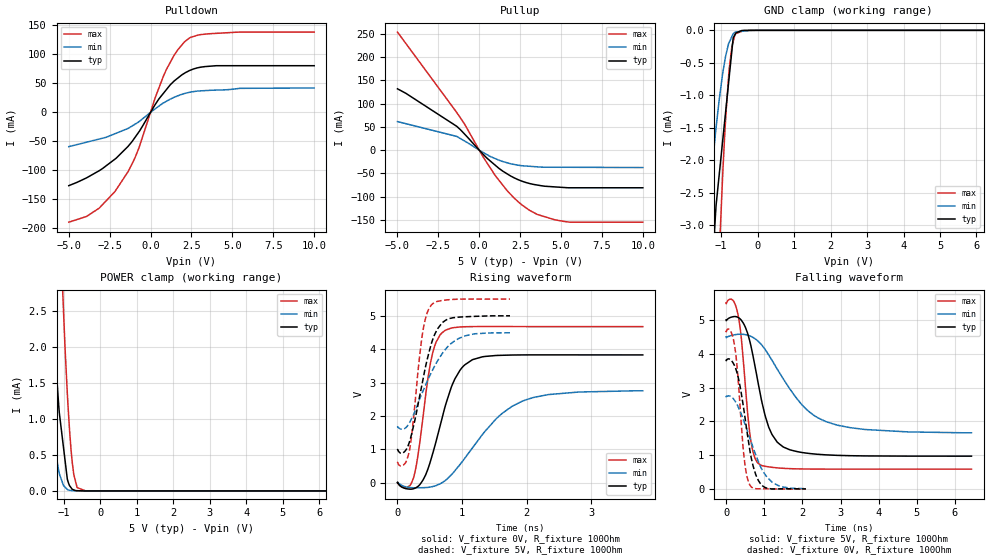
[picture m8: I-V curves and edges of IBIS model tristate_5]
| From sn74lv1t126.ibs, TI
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|   tristate_5 Model
[Model]   tristate_5
Model_type   3-state
Polarity   Non-Inverting
Vmeas = 2.5
Vref = 0
Cref = 30pF
Rref = 100
|   typ   min   max
|   (nom PVT)   (fast PVT)   (slow PVT)
C_comp   2.245e-12   2.225e-12   2.269e-12
| Where nom  PVT is Nominal Process, 5V, 40C
|   Fast PVT is Strong Process,  5.5V, -40C
|   Slow PVT is Weak Process,   4.5V, 140C
[Voltage Range]   5   4.5   5.5
|Junction Temperature
[Temperature Range]   40   140   -40
[Pullup Reference]   5   4.5   5.5
[Pulldown Reference]   0   0   0
[Power Clamp Reference]   5   4.5   5.5
[GND Clamp Reference]   0   0   0
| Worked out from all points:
|   slope of the pulldown table from 0 to 0.75 V, typ, clamps not added: 23.8 ohm
|   slope of the pullup table from 0 to 0.75 V, typ, clamps not added: 29.4 ohm
|   GND clamp passes 1 mA (typ) near -0.83 V on its own axis
|   POWER clamp passes 1 mA (typ) near -1.10 V on its own axis
|   falling waveform, V_fixture 5V, R_fixture 100Ohm: 20-80 % time 480ps typ, 1.11ns min, 237ps max; typ from 5 V to 0.975 V
|   rising waveform, V_fixture 0V, R_fixture 100Ohm: 20-80 % time 348ps typ, 740ps min, 202ps max; typ from 0 V to 3.83 V
|   rising waveform, V_fixture 5V, R_fixture 100Ohm: 20-80 % time 270ps typ, 425ps min, 163ps max; typ from 0.975 V to 5 V
|   falling waveform, V_fixture 0V, R_fixture 100Ohm: 20-80 % time 328ps typ, 548ps min, 195ps max; typ from 3.83 V to 0.009 V
[Pulldown]
|   Voltage   I(typ)   I(min)   I(max)
-5V       -126.6mA   -59.23mA   -189.6mA
-3.905V   -113mA     -51.53mA   -179.6mA
-3.14V    -100.8mA   -46.15mA   -165.3mA
-2.189V   -81.04mA   -37.15mA   -137mA
-1.375V   -58.76mA   -27.86mA   -102.5mA
-709.5mV  -33.68mA   -16.18mA   -61.28mA
302.5mV   14.21mA    6.321mA    26.75mA
803mV     33.33mA    16.31mA    63.51mA
1.419V    53.33mA    25.57mA    97.38mA
2.145V    68.57mA    32.8mA     123.1mA
3.547V    79.25mA    37.69mA    135.4mA
10V       80.29mA    41.89mA    138.3mA
[GND Clamp]
|   Voltage   I(typ)   I(min)   I(max)
-5V       -79.76mA   -44.68mA   -116.9mA
-1.375V   -5.076mA   -2.914mA   -8.957mA
-1.255V   -3.79mA    -2.182mA   -6.711mA
-1.157V   -2.846mA   -1.586mA   -5.027mA
-1.05V    -2.206mA   -1.056mA   -3.423mA
-963mV    -1.726mA   -683.2uA   -2.291mA
-877.5mV  -1.256mA   -396.8uA   -1.369mA
-786.5mV  -756.1uA   -193.2uA   -640.4uA
-704mV    -303uA     -93.82uA   -242.6uA
-670mV    -116.2uA   -53.23uA   -171.9uA
-616.5mV  -62.01uA   -27.22uA   -60.64uA
10V       0A         0A         0A
[Pullup]
|   Voltage   I(typ)   I(min)   I(max)
-5V       132mA      61.56mA    253.9mA
-4.5V     122.6mA    57.15mA    230.1mA
-1.375V   51.32mA    29.6mA     81.04mA
-858mV    33.19mA    18.98mA    53.77mA
265mV     -9.864mA   -5.349mA   -15.98mA
968mV     -32.02mA   -17.94mA   -53.99mA
1.788V    -52.63mA   -27.86mA   -90.19mA
2.635V    -66.91mA   -33.47mA   -118.3mA
3.547V    -74.93mA   -35.76mA   -138.1mA
4.631V    -78.93mA   -36.67mA   -149.7mA
5.192V    -80.23mA   -36.69mA   -153.2mA
10V       -80.78mA   -37.35mA   -154.8mA
[POWER Clamp]
|   Voltage   I(typ)   I(min)   I(max)
-5V       81.69mA    45.06mA    132.8mA
-1.735V   7.225mA    3.528mA    16.16mA
-1.373V   3.058mA    1.094mA    8.26mA
-1.27V    2.158mA    682.3uA    6.386mA
-1.125V   1.09mA     243.3uA    4.061mA
-1.067V   846.4uA    157.9uA    3.223mA
-1.008V   598.9uA    73.93uA    2.494mA
-850.5mV  81.54uA    9.359uA    905.1uA
-726mV    14.49uA    3.161uA    225.7uA
-632.5mV  3.405uA    656.9nA    46.34uA
-401.5mV  48.63nA    305.4nA    305.7nA
10V       0A         0A         0A
[Ramp]
R_load = 100
|   typ   min   max
dV/dt_r   2.29631/3.48301e-10   1.65453/7.38171e-10   2.80548/2.01165e-10
dV/dt_f   2.41476/4.76742e-10   1.70472/1.10947e-09   2.94472/2.36728e-10
[Falling Waveform]
V_fixture = 5V
V_fixture_min = 4.5V
V_fixture_max = 5.5V
R_fixture = 100Ohm
|   Time   V(typ)   V(min)   V(max)
0s        5V         4.5V       5.5V
172ps     5.09V      4.549V     5.585V
314ps     5.074V     4.574V     5.147V
640ps     4.282V     4.517V     1.49V
902ps     2.774V     4.299V     717.3mV
1.114ns   1.84V      3.967V     659.6mV
1.338ns   1.392V     3.55V      630.3mV
2.018ns   1.079V     2.457V     597.1mV
2.604ns   1.015V     2.001V     592.9mV
6.434ns   975.5mV    1.665V     592.1mV
[Rising Waveform]
V_fixture = 0V
V_fixture_min = 0V
V_fixture_max = 0V
R_fixture = 100Ohm
|   Time   V(typ)   V(min)   V(max)
0s        997pV      9.968nV    1.769nV
146ps     -188mV     -136.3mV   -148.9mV
250ps     -184.7mV   -156.4mV   148.6mV
518ps     687.7mV    -130.8mV   3.652V
598ps     1.236V     -90.43mV   4.212V
736ps     2.268V     54.71mV    4.559V
1.044ns   3.532V     733.4mV    4.672V
1.538ns   3.811V     1.93V      4.678V
1.92ns    3.827V     2.43V      4.677V
3.798ns   3.827V     2.751V     4.676V
[Rising Waveform]
V_fixture = 5V
V_fixture_min = 4.5V
V_fixture_max = 5.5V
R_fixture = 100Ohm
|   Time   V(typ)   V(min)   V(max)
0s        975.4mV    1.659V     592.1mV
118ps     944.8mV    1.628V     575.8mV
188ps     1.234V     1.799V     982.9mV
228ps     1.529V     1.952V     1.549V
378ps     2.923V     2.666V     4.348V
448ps     3.589V     2.984V     5.014V
518ps     4.12V      3.275V     5.306V
692ps     4.791V     3.864V     5.46V
954ps     4.961V     4.326V     5.499V
1.742ns   5V         4.489V     5.501V
[Falling Waveform]
V_fixture = 0V
V_fixture_min = 0V
V_fixture_max = 0V
R_fixture = 100Ohm
|   Time   V(typ)   V(min)   V(max)
0s        3.827V     2.758V     4.676V
114ps     3.826V     2.742V     4.672V
226ps     3.637V     2.616V     4.207V
300ps     3.376V     2.47V      3.446V
466ps     2.342V     2.008V     990.9mV
616ps     1.193V     1.527V     136.1mV
776ps     434.3mV    1.016V     15.73mV
984ps     73.5mV     496.3mV    13.66mV
1.346ns   7.055mV    116.6mV    6.101mV
2.092ns   9.389mV    17.98mV    742.3uV
